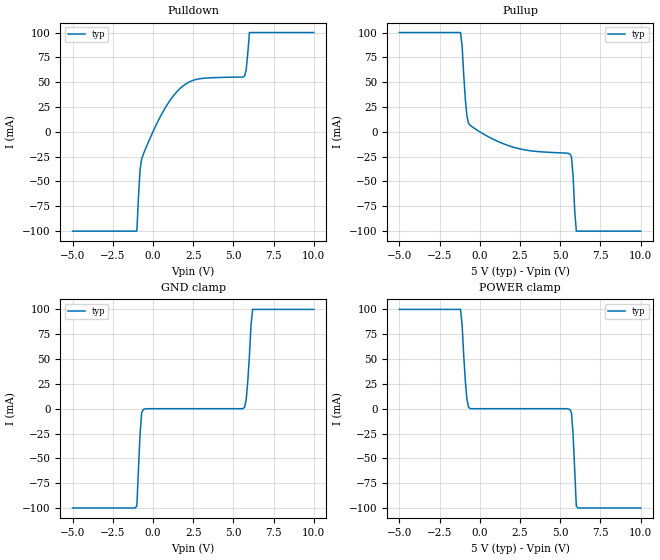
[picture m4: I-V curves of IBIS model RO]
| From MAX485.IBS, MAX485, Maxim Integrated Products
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|   Driver Receiver 3-State Output RO
[Model]   RO
|Signals   R0
Model_type   3-state
Polarity   Non-Inverting
C_comp   0.538pF   NA   NA
[Temperature Range]   25   -40   85
[Voltage Range]   5.00V   4.75V   5.25V
[Pullup Reference]   5.00V   4.75V   5.25V
[Pulldown Reference]   0.00V   0.00V   0.00V
[POWER Clamp Reference]   5.00V   4.75V   5.25V
[GND Clamp Reference]   0.00V   0.00V   0.00V
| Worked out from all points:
|   slope of the pulldown table from 0 to 0.75 V, typ, clamps not added: 31.6 ohm
|   slope of the pullup table from 0 to 0.75 V, typ, clamps not added: 110 ohm
|   GND clamp passes 1 mA (typ) near -0.61 V on its own axis
|   POWER clamp passes 1 mA (typ) near -0.66 V on its own axis
[Pullup]
| Note that the[Pulldown]voltage table is referenced to Vcc
| and is calculated using Vtable=Vcc - Vmeasured.
| Also, the Semiconductor Parameter Analyzer (Force and Sense)
| clamps the supply current to 100mA to protect the system.
| V(V)  I(typ)   I(min)  I(max)
-5V       100mA      NA         NA
-1.2V     100mA      NA         NA
-1.1V     86.68mA    NA         NA
-900mV    32.81mA    NA         NA
-800mV    15.84mA    NA         NA
-600mV    6.545mA    NA         NA
2.1V      -15.53mA   NA         NA
5.6V      -22.29mA   NA         NA
5.7V      -25.17mA   NA         NA
5.8V      -44.46mA   NA         NA
6V        -100mA     NA         NA
10V       -100mA     NA         NA
[Pulldown]
| Note that the[Pulldown]voltage table is referenced to Gnd.
| Also, the Semiconductor Parameter Analyzer (Force and Sense)
| clamps the supply current to 100mA to protect the system.
| V(V)  I(typ)   I(min)  I(max)
-5V       -100mA     NA         NA
-1V       -100mA     NA         NA
-900mV    -66.08mA   NA         NA
-800mV    -38.15mA   NA         NA
-700mV    -27.28mA   NA         NA
600mV     19.46mA    NA         NA
1.8V      45.24mA    NA         NA
2.9V      53.4mA     NA         NA
5.7V      56.27mA    NA         NA
5.8V      62.75mA    NA         NA
6V        100mA      NA         NA
10V       100mA      NA         NA
[POWER_clamp]
| Note that the[POWER_clamp]voltage table is referenced to Vcc
| and is calculated using Vtable=Vcc - Vmeasured.
| Also, the Semiconductor Parameter Analyzer (Force and Sense)
| clamps the supply current to 100mA to protect the system.
| V(V)  I(typ)   I(min)  I(max)
-5V       100mA      NA         NA
-1.2V     100mA      NA         NA
-1.1V     84.39mA    NA         NA
-900mV    27.9mA     NA         NA
-800mV    9.474mA    NA         NA
-600mV    102.8uA    NA         NA
5.6V      -798.6uA   NA         NA
5.7V      -4.22mA    NA         NA
5.8V      -25.83mA   NA         NA
6V        -97.91mA   NA         NA
6.1V      -100mA     NA         NA
10V       -100mA     NA         NA
[GND_clamp]
| Note that the[GND_clamp]voltage table is referenced to Gnd.
| Also, the Semiconductor Parameter Analyzer (Force and Sense)
| clamps the supply current to 100mA to protect the system.
| V(V)  I(typ)   I(min)  I(max)
-5V       -100mA     NA         NA
-1.1V     -100mA     NA         NA
-1V       -97.92mA   NA         NA
-800mV    -25.82mA   NA         NA
-700mV    -4.222mA   NA         NA
-600mV    -798.3uA   NA         NA
5.6V      102.7uA    NA         NA
5.8V      9.473mA    NA         NA
5.9V      27.89mA    NA         NA
6.1V      84.39mA    NA         NA
6.2V      100mA      NA         NA
10V       100mA      NA         NA
[Ramp]
| variable   typ   min   max
dV/dt_r   3.12/17.6nS   NA   NA
dV/dt_f   3.10/2.89nS   NA   NA
R_load = 5Kohms
|End [Model] RO
